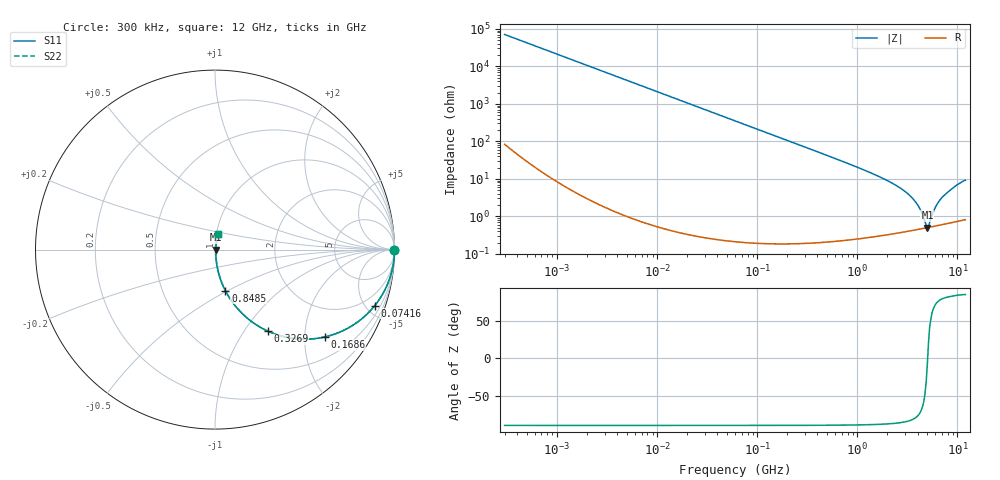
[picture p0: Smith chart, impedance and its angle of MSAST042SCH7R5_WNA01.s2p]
! MSAST042SCH7R5_WNA01  S-PARAMETER MODEL  ( General Type )
! Model Generated by TAIYO YUDEN Corporation (http://www.ty-top.com)
! Version 1.0
! TAIYO YUDEN Control No. 150820
! Copyright(c) 2015 TAIYO YUDEN CO.,LTD. All Rights Reserved.
! Product Description (link to TY-COMPAS)
! https://ds.yuden.co.jp/TYCOMPAS/or/detail?pn=MSAST042SCH7R5BWNA01&u=M
! Products Name : Multilayer Ceramic Capacitors
! Characteristics :
!  Capacitance : 7.5 pF , Rated Voltage : 25V , TCC : CH / C0H
!  Case Size : 0.4 x 0.2 / 0.016 x 0.008 [mm/inch] , Thickness : 0.2 / 0.008 [mm/inch]
!  (Conditions: Temperature = 25 degC , DC Bias Current/Voltage = 0A / 0V)
! External Node Assignments :
!  1  o---| |---o  2
! GND o---------o GND
! Frequency Range : 0.3MHz  -  12000MHz  [ 401 STEP ]
# MHz S RI R 50
! Freq[MHz].  S11 Real  S11 Imag  S21 Real  S21 Imag  S12 Real  S12 Imag  S22 Real  S22 Imag
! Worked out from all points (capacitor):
!   401 points, 300 kHz to 12 GHz, reference 50 ohm
!   read as one part in series: C = 7.5 pF near 316.3 kHz
!   lowest |Z| = 504 mohm at 5.006 GHz (marker M1)
!   series resonance near 5.039 GHz, so ESL is about 130 pH
!   S11 on the Smith chart (normalised r, x): 300 kHz: open; 74.16 MHz: 1.00, -5.72; 168.6 MHz: 1.00, -2.51; 326.9 MHz: 1.00, -1.29; 848.5 MHz: 1.00, -0.49; 12 GHz: 1.02, +0.18
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0.3  1 -0.00141  3.67e-06 0.00141  3.67e-06 0.00141  1 -0.00141
1.769972  0.9999 -0.00835  7.21e-05 0.00835  7.21e-05 0.00835  0.9999 -0.00835
10.44266  0.9976 -0.0491  0.00243 0.0491  0.00243 0.0491  0.9976 -0.0491
27.10171  0.9839 -0.1257  0.0161 0.1257  0.0161 0.1257  0.9839 -0.1257
60  0.9257 -0.2619  0.0743 0.2619  0.0743 0.2619  0.9257 -0.2619
74.16388  0.8908 -0.3115  0.1092 0.3115  0.1092 0.3115  0.8908 -0.3115
168.5979  0.612 -0.4866  0.388 0.4866  0.388 0.4866  0.612 -0.4866
326.9496  0.2949 -0.4545  0.7051 0.4545  0.7051 0.4545  0.2949 -0.4545
353.9943  0.2629 -0.4386  0.7371 0.4386  0.7371 0.4386  0.2629 -0.4386
540.8523  0.132 -0.3357  0.868 0.3357  0.868 0.3357  0.132 -0.3357
848.5281  0.0577 -0.2283  0.9423 0.2283  0.9423 0.2283  0.0577 -0.2283
2088.533  0.0102 -0.083  0.9898 0.083  0.9898 0.083  0.0102 -0.083
2870.14  0.00624 -0.0495  0.9938 0.0495  0.9938 0.0495  0.00624 -0.0495
3642.919  0.005 -0.0276  0.995 0.0276  0.995 0.0276  0.005 -0.0276
4158.869  0.00479 -0.0162  0.9952 0.0162  0.9952 0.0162  0.00479 -0.0162
4747.894  0.00486 -0.00511  0.9951 0.00511  0.9951 0.00511  0.00486 -0.00511
5006.236  0.00497 -0.000635  0.995 0.000635  0.995 0.000635  0.00497 -0.000635
5278.635  0.00513 0.00454  0.9949 -0.00454  0.9949 -0.00454  0.00513 0.00454
6026.253  0.00576 0.0166  0.9942 -0.0166  0.9942 -0.0166  0.00576 0.0166
6879.757  0.00675 0.0291  0.9932 -0.0291  0.9932 -0.0291  0.00675 0.0291
9454.42  0.0109 0.0617  0.9891 -0.0617  0.9891 -0.0617  0.0109 0.0617
12000  0.0161 0.0889  0.9839 -0.0889  0.9839 -0.0889  0.0161 0.0889
